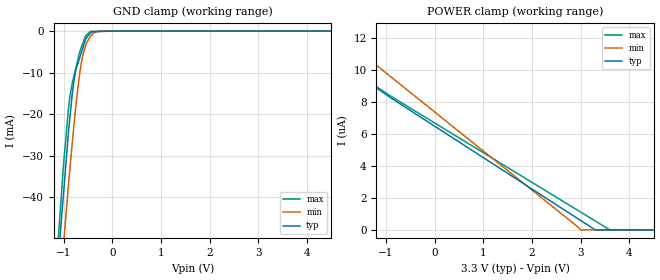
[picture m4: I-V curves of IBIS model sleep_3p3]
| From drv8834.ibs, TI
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|   sleep_3p3 Model
[Model]   sleep_3p3
Model_type   Input
Vinl = 0.7
Vinh = 2
|   typ   min   max
|   (nom PVT)   (fast PVT)   (slow PVT)
|C_comp from frequency sweep method (F=250KHz)
|Average
|C_comp   2.715e-12   2.495e-12   2.942e-12
|C_comp from LC tank measurement(L=1nH)
|Average
|Resonant Frequency(Hz)   4.340e+09   4.370e+09   4.270e+09
 C_comp   1.346e-12   1.328e-12   1.391e-12
| Where nom  PVT is Nominal Process, 3.3V, 27C
|   Fast PVT is Strong Process,  3.6V, -40C
|   Slow PVT is Weak Process,   3V, 125C
[Voltage Range]   3.3   3   3.6
|Ambient Temperature   25   150   -40
|Junction Temperature
[Temperature Range]   27   125   -40
[Power Clamp Reference]   3.3   3   3.6
[GND Clamp Reference]   0   0   0
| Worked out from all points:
|   GND clamp passes 1 mA (typ) near -0.49 V on its own axis
[GND Clamp]
|   Voltage   I(typ)   I(min)   I(max)
-3.3V     -460.7mA   -437.6mA   -483mA
-1.166V   -65.08mA   -75.53mA   -59.75mA
-1.065V   -48.71mA   -60.47mA   -42.9mA
-1.001V   -39.18mA   -51.41mA   -32.23mA
-896.4mV  -24.03mA   -36.69mA   -18.28mA
-782.1mV  -11.67mA   -22.16mA   -10.59mA
-690mV    -7.213mA   -12.1mA    -6.103mA
-633mV    -5.106mA   -7.541mA   -3.836mA
-531mV    -1.656mA   -2.971mA   -1.02mA
-453.6mV  -536.3uA   -1.304mA   -110.9uA
-3mV      0A         -14.67nA   0A
6.6V      0A         0A         0A
[POWER Clamp]
|   Voltage   I(typ)   I(min)   I(max)
-3.3V     43.26uA    15.44uA    48.34uA
-3V       12.7uA     14.71uA    12.56uA
-897.6mV  8.25uA     9.564uA    8.355uA
2.814V    955.3nA    500.5nA    1.46uA
2.997V    595.7nA    0A         1.12uA
3.297V    0A         0A         563.4nA
3.596V    0A         0A         0A
6.6V      0A         0A         0A
